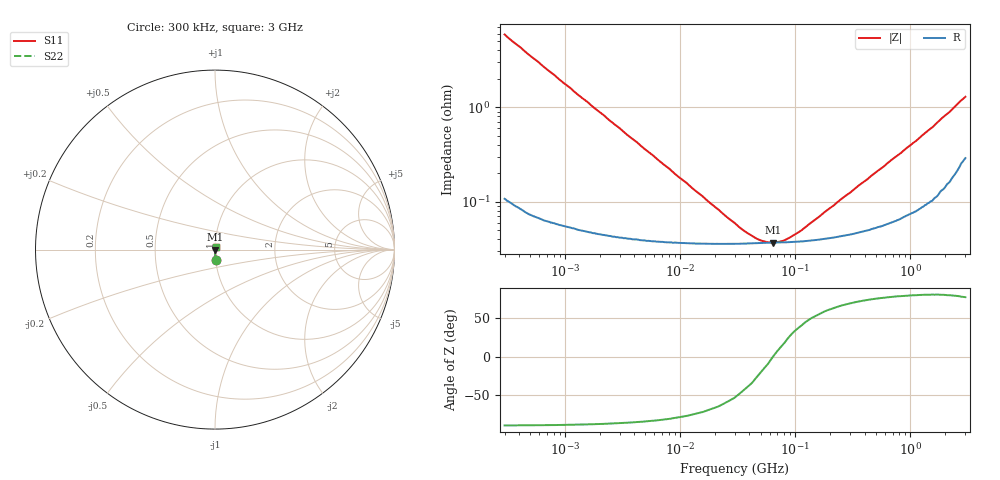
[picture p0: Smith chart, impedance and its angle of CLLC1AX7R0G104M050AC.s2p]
! S-Parameter Data Generated by TDK Corporation
! Copyright(C) 2022 TDK Corporation.
! All Rights Reserved.
! TDK P/N: CLLC1AX7R0G104M050AC (Multilayer Ceramic Chip Capacitor)
! Property: C=100nF
! Size(LxWxT): 1.6x0.8x0.5mm
! Model Type: s2p (Touchstone File Format Version 1.0)
! Frequency: DC=Yes Start=0.3MHz Stop=3000MHz 402points Log-sweep
! Model Generated on Apr. 15, 2022
! Port Assignments:
!  1 ---| |--- 2
! Applicable Conditions:
!  Temperature = 25 degC
!  DC Bias Voltage = 0 V
!  Small Signal Operation
! Terms and conditions regarding TDK Simulation Models
! (1)This simulation model is being provided solely for informational purposes. Please refer to the specifications of the products in terms of detailed characteristics of such products.
! (2)In no event shall TDK Corporation of any of its subsidiaries be liable for any loss or damage arising, directly or indirectly,
!  From any information contained in this simulation model, including, but not limited to loss or damages arising from any inaccuracies, omissions or errors in connection with such information.
! (3)Any and all copyrights on this simulation model are owned by TDK Corporation.
!  Duplication or redistribution of this simulation model without prior written permission from TDK Corporation is prohibited.
! (4)This simulation model is subject to any modification or change without any prior notice.
! (5)Neither TDK Corporation nor any of its subsidiaries shall make any warranty, express or implied,
!  Including but not limited to the correctness, implied warranties of merchantability and fitness for a particular purpose with respect to this simulation models.
! (6)The use of this simulation model shall be deemed to have consented to the terms and conditions hereof.
# Hz S MA R 50
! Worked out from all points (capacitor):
!   401 points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, 300 kHz to 3 GHz, reference 50 ohm
!   read as one part in series: C = 90.7 nF near 314.1 kHz
!   lowest |Z| = 37.1 mohm at 64.14 MHz (marker M1)
!   series resonance near 64.11 MHz, so ESL is about 68 pH
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300000  0.05875 -85.6  0.9972 3.4  0.9972 3.4  0.05875 -85.6
404689  0.04371 -86.4  0.9982 2.5  0.9982 2.5  0.04371 -86.4
641389  0.02741 -87.1  0.999 1.6  0.999 1.6  0.02741 -87.1
1403210  0.01261 -87.0  0.9994 0.7  0.9994 0.7  0.01261 -87.0
6563280  0.002725 -81.9  0.9996 0.2  0.9996 0.2  0.002725 -81.9
1.11461e7  0.001619 -76.9  0.9996 0.1  0.9996 0.1  0.001619 -76.9
3e7  0.0005928 -52.6  0.9996 0.0  0.9996 0.0  0.0005928 -52.6
3.60679e7  0.0004923 -42.8  0.9996 0.0  0.9996 0.0  0.0004923 -42.8
4.64645e7  0.0004065 -26.1  0.9996 0.0  0.9996 0.0  0.0004065 -26.1
5.4591e7  0.0003791 -13.8  0.9996 0.0  0.9996 0.0  0.0003791 -13.8
6.41389e7  0.0003707 0.0  0.9996 -0.0  0.9996 -0.0  0.0003707 0.0
7.53566e7  0.000382 13.0  0.9996 -0.0  0.9996 -0.0  0.000382 13.0
8.65209e7  0.0004091 23.9  0.9996 -0.0  0.9996 -0.0  0.0004091 23.9
1.11461e8  0.0004921 39.5  0.9996 -0.0  0.9996 -0.0  0.0004921 39.5
1.40321e8  0.0006132 50.4  0.9996 -0.0  0.9996 -0.0  0.0006132 50.4
5.71638e8  0.002305 75.9  0.9994 -0.1  0.9994 -0.1  0.002305 75.9
6.56328e8  0.002662 77.0  0.9994 -0.1  0.9994 -0.1  0.002662 77.0
1.11461e9  0.004391 79.4  0.9992 -0.2  0.9992 -0.2  0.004391 79.4
1.53858e9  0.006085 80.0  0.999 -0.3  0.999 -0.3  0.006085 80.0
2.22393e9  0.009099 78.9  0.9983 -0.5  0.9983 -0.5  0.009099 78.9
2.73603e9  0.0117 77.0  0.9974 -0.7  0.9974 -0.7  0.0117 77.0
3e9  0.01287 76.3  0.997 -0.7  0.997 -0.7  0.01287 76.3
